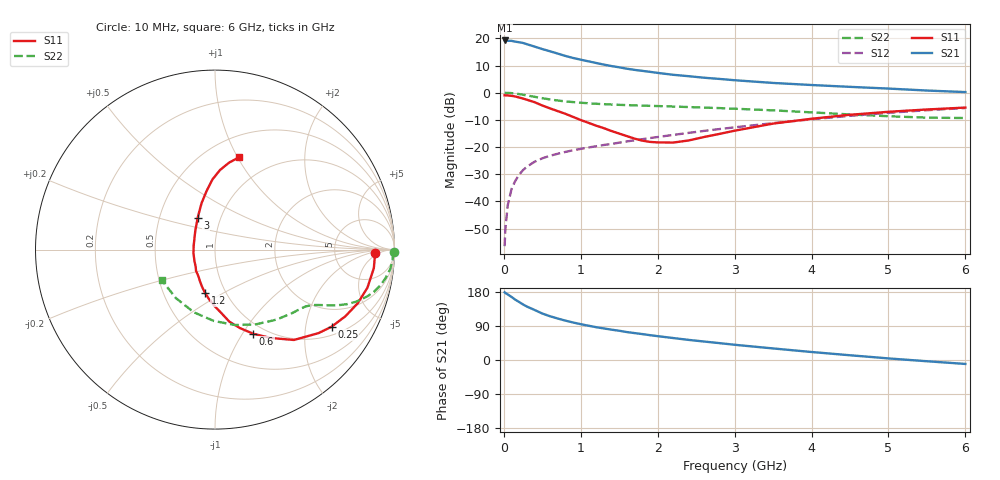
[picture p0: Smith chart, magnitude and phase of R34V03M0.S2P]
! SIEMENS Small Signal Semiconductors
! BFR181
! Si NPN RF Bipolar Junction Transistor in SOT23
! VCE = 4 V  IC = 3 mA
! Common Emitter S-Parameters:  May  1996
# GHz  S  MA  R  50
!  f  S11  S21  S12  S22
! GHz  MAG  ANG  MAG  ANG  MAG  ANG  MAG  ANG
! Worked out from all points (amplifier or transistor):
!   36 points, 10 MHz to 6 GHz, reference 50 ohm
!   highest |S21| = 19.2 dB at 10 MHz (marker M1)
!   |S21| within 3 dB of that: start of sweep to 481.6 MHz
!   unconditionally stable (mu >= 1): 1.37 GHz to 3.217 GHz
!   at 250 MHz: K = 0.30, MSG = 23.4 dB, |S12| = -28.5 dB
!   at 1.4 GHz: K = 1.01, MAG = 13.7 dB, |S12| = -18.9 dB
!   at 6 GHz: K = 0.86, MSG = 2.9 dB, |S12| = -5.6 dB
!   lowest NFmin = 1.40 dB at 450 MHz
!   S11 on the Smith chart (normalised r, x): 10 MHz: 17, -3; 250 MHz: 1.28, -2.79; 600 MHz: 0.88, -1.12; 1.2 GHz: 0.80, -0.41; 3 GHz: 0.78, +0.28; 6 GHz: 0.71, +1.02
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0.01  0.8939 -1.3  9.139 178.6  0.0015 92.9  0.995 -0.7
0.02  0.8912 -2.8  9.042 176.9  0.0031 85.0  0.9914 -1.4
0.05  0.8909 -6.7  9.006 173.1  0.0084 86.8  0.9916 -3.3
0.1  0.8755 -14.0  8.989 166.4  0.0169 81.4  0.9816 -6.5
0.15  0.8497 -20.6  8.684 159.0  0.024 77.8  0.9621 -9.7
0.25  0.7787 -33.5  8.214 146.5  0.0377 71.5  0.917 -14.8
0.3  0.7411 -38.9  7.798 141.0  0.0435 69.3  0.8888 -17.0
0.4  0.6682 -48.9  7.043 132.0  0.0537 65.1  0.8396 -20.2
0.5  0.5808 -57.9  6.347 122.6  0.062 62.3  0.7928 -22.6
0.6  0.5146 -65.6  5.778 115.5  0.069 60.3  0.7504 -24.4
0.7  0.4586 -72.4  5.242 109.5  0.0752 59.8  0.7177 -25.7
0.8  0.4088 -78.8  4.744 103.9  0.0813 58.3  0.6914 -26.6
0.9  0.3584 -83.9  4.353 99.0  0.0873 58.0  0.6717 -27.4
1.1  0.2786 -96.8  3.774 90.5  0.098 58.0  0.6387 -28.9
1.2  0.2472 -103.0  3.517 86.6  0.1034 58.5  0.6253 -29.7
1.6  0.1588 -131.6  2.759 73.7  0.1269 59.4  0.5911 -32.8
2.2  0.1209 169.1  2.135 58.0  0.167 59.4  0.5561 -39.6
3  0.1998 119.2  1.695 40.2  0.2305 56.9  0.5069 -51.5
3.5  0.2698 106.1  1.511 30.5  0.2749 53.8  0.473 -61.9
4.5  0.392 92.0  1.28 12.5  0.3753 44.5  0.3978 -90.9
5.5  0.4908 80.8  1.095 -3.3  0.476 32.1  0.3472 -128.9
6  0.5324 75.3  1.026 -10.4  0.5221 24.9  0.3418 -149.8
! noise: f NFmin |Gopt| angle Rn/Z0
0.45  1.4  0.56  17  0.36
0.9  1.5  0.45  35  0.34
1.8  1.85  0.25  82  0.36
